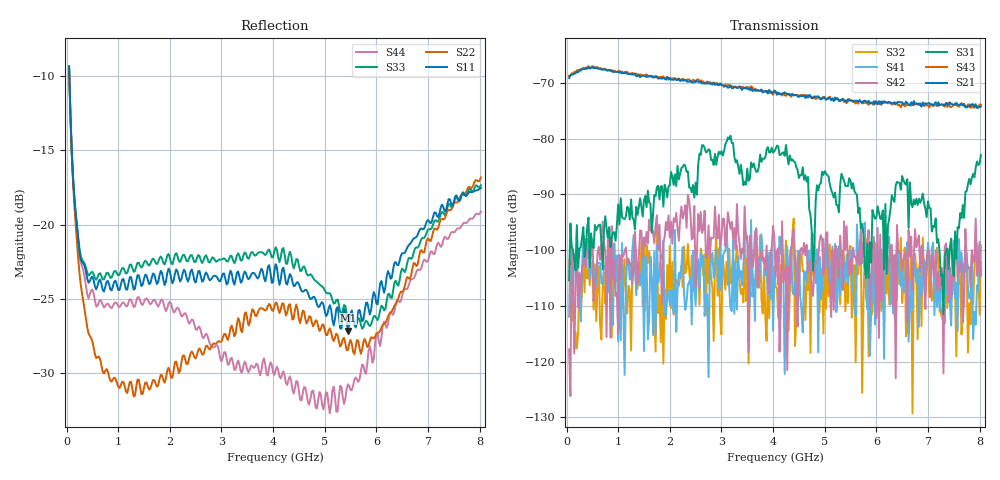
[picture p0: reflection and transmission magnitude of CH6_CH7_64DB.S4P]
!Agilent Technologies,E5071C,MY46316741,A.11.02
!Date: Mon Jun 01 10:35:53 2026
!Data & Calibration Information:
!1:CH6 INPUT 2:CH6 OUTPUT 3:CH7 INPUT 4:CH7 OUTPUT
!Freq	S11:SOLT4(ON)	S12:SOLT4(ON)	S13:SOLT4(ON)	S14:SOLT4(ON)
!	S21:SOLT4(ON)	S22:SOLT4(ON)	S23:SOLT4(ON)	S24:SOLT4(ON)
!	S31:SOLT4(ON)	S32:SOLT4(ON)	S33:SOLT4(ON)	S34:SOLT4(ON)
!	S41:SOLT4(ON)	S42:SOLT4(ON)	S43:SOLT4(ON)	S44:SOLT4(ON)
!PortZ  Port1:50+j0  Port2:50+j0  Port3:50+j0  Port4:50+j0
!Above PortZ is port z conversion or system Z0 setting when saving the data.
!When reading, reference impedance value at option line is always used.
# Hz S dB R 50
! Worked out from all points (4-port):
!   320 points, 50 MHz to 8.025 GHz, reference 50 ohm
!   strongest paths, dB at 50 MHz, 2.05 GHz, 4.05 GHz, 6.05 GHz, 8.025 GHz:
!     S21: -69.1, -69.4, -71.5, -73.3, -74.2
!     S43: -68.7, -69.3, -71.7, -73.8, -73.9
!     S31: -105.4, -86.8, -81.8, -93.3, -82.9
!     S42: -117.8, -98.9, -104.9, -115.8, -104.6
!     S41: -111.9, -107.2, -103.3, -107.0, -104.4
!     S32: -101.8, -102.2, -106.6, -112.6, -99.1
!   lowest |S11| = -27.1 dB at 5.45 GHz (marker M1), VSWR 1.09, Z = 48.2 - j3.94 ohm
!   |S11| at or under -10 dB: 55.3 MHz to end of sweep
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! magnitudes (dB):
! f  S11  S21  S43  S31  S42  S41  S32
! 50 MHz  -9.3  -69.1  -68.7  -105.4  -117.8  -111.9  -101.8
! 125 MHz  -16.8  -68.5  -68.3  -100.0  -105.3  -109.4  -104.7
! 275 MHz  -22.3  -67.8  -67.5  -99.5  -107.7  -112.8  -110.9
! 850 MHz  -24.4  -67.8  -67.7  -99.5  -115.7  -104.1  -99.3
! 4.2 GHz  -22.9  -71.9  -71.8  -82.5  -105.9  -103.9  -104.6
! 5.45 GHz  -27.1  -72.9  -73.3  -88.5  -102.1  -106.3  -109.5
! 8.025 GHz  -17.5  -74.2  -73.9  -82.9  -104.6  -104.4  -99.1
